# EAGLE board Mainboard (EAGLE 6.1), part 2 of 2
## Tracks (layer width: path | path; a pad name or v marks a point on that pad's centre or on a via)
!MOT0_FLAG  (via drill 0.6)
  Sig1 0.254: U$2.24 42.48,56.77 v42.86,57.15
  Sig1 0.406: U$3.31 74.36,23.88 v74.61,24.13 | v64.77,45.72 64.77,41.91 68.58,38.1 72.39,38.1 75.25,35.24 v75.25,31.11
  Sig2 0.406: v74.61,24.13 76.2,25.72 76.2,30.16 v75.25,31.11
  Bottom_GND 0.406: v42.86,57.15 42.86,49.21 43.18,48.9 60.01,48.9 62.87,46.04 64.45,46.04 v64.77,45.72
!MOT1_FLAG  (via drill 0.6)
  Sig1 0.254: U$2.23 41.39,57.27 v41.91,57.78
  Sig1 0.406: U$4.31 99.76,23.88 v100.17,24.29 | v100.01,30.8 97.79,33.02 97.79,35.56 96.2,37.15 87.95,37.15 87.63,37.47 74.93,37.47 73.03,39.37 69.22,39.37 67.31,41.27 v67.31,43.81
  Bottom_GND 0.406: v100.17,24.29 100.17,24.61 101.6,26.04 101.6,29.21 v100.01,30.8 | v41.91,57.78 41.91,49.21 42.86,48.26 59.69,48.26 62.55,45.4 63.5,45.4 64.14,44.77 66.36,44.77 v67.31,43.81
!MOT2_FLAG  (via drill 0.6)
  Sig1 0.305: U$2.16 37.21,59.75 v37.15,59.69
  Sig1 0.406: U$5.31 125.16,23.88 v125.41,24.13
  Sig2 0.406: v125.41,24.13 126.84,25.72 127,30.48 v126.36,31.11
  Bottom_GND 0.406: v37.15,59.69 37.15,49.21 41.27,45.09 58.1,45.09 61.59,41.59 86.68,41.59 90.81,37.47 95.89,37.47 100.65,32.7 106.68,32.7 107.95,31.43 126.05,31.43 v126.36,31.11
!MOT3_FLAG  (via drill 0.6)
  Sig1 0.305: U$2.15 37.71,60.72 v38.1,60.33
  Sig1 0.406: U$6.31 149.92,23.88 v150.18,24.13
  Sig2 0.406: v150.18,24.13 150.18,24.45 151.45,25.72 151.45,29.21 v148.91,31.75
  Bottom_GND 0.406: v38.1,60.33 38.1,49.21 41.59,45.72 58.42,45.72 61.91,42.23 87,42.23 91.12,38.1 96.2,38.1 100.97,33.34 107,33.34 107.63,32.7 147.96,32.7 v148.91,31.75
!MOT4_FLAG  (via drill 0.6)
  Sig1 0.305: U$2.60 49.37,58.27 v49.85,57.78
  Sig1 0.406: U$7.31 137.06,51.82 v137.48,52.23
  Bottom_GND 0.406: v49.85,57.78 49.85,57.15 56.83,50.16 60.64,50.16 63.5,47.31 65.41,47.31 66.67,46.04 66.99,46.04 67.31,45.72 67.63,45.72 69.22,44.13 87,44.13 87.95,45.09 87.95,57.78 89.53,59.37 137.79,59.37 139.06,58.1 139.06,54.93 137.48,53.34 v137.48,52.23
!MOT5_FLAG  (via drill 0.6)
  Sig1 0.305: U$2.59 48.28,57.77 v48.9,57.15
  Sig1 0.406: U$8.31 111.03,51.82 111.76,52.55 112.55,52.55 113.51,53.5 v113.82,53.5
  Bottom_GND 0.406: v48.9,57.15 56.52,49.53 60.33,49.53 63.18,46.67 65.09,46.67 66.36,45.4 66.67,45.4 66.99,45.09 67.31,45.09 68.9,43.5 87.95,43.5 88.9,44.45 88.9,48.9 89.53,49.53 92.71,49.53 93.66,50.48 93.66,51.75 96.2,54.29 112.87,54.29 v113.82,53.5
!MOT_RESET  (via drill 0.6)
  Sig1 0.406: U$3.6 56.26,23.88 v55.88,23.5 | v78.11,31.75 v81.28,31.75 | v103.82,31.75 v106.36,31.75 | v131.13,31.75 v128.59,31.75 120.33,40.01 v119.7,40.01 | U$4.6 82.3,23.88 v81.92,23.5 | U$5.6 108.01,23.88 v107.63,23.5 | U$6.6 131.83,23.88 v131.44,23.5 | U$7.6 119.92,51.82 119.38,51.28 v119.38,50.8 | U$8.6 95.31,51.82 v94.61,51.12
  Sig2 0.406: v55.88,23.5 55.88,29.84 58.1,32.07 77.79,32.07 v78.11,31.75 | v103.82,31.75 103.19,32.07 81.6,32.07 v81.28,31.75 81.28,24.13 v81.92,23.5 | v128.59,31.75 128.27,32.07 106.68,32.07 v106.36,31.75 106.36,24.77 v107.63,23.5 | v131.13,31.75 131.44,31.43 v131.44,23.5
  Bottom_GND 0.406: v119.38,50.8 119.06,50.48 117.47,50.48 115.57,48.42 115.57,43.18 | 115.57,43.18 118.75,40.01 v119.7,40.01 | v94.61,51.12 94.61,49.85 95.89,48.58 95.89,41.59 98.11,39.37 111.76,39.37 115.57,43.18
!SPI_CS  (via drill 0.6)
  Sig1 0.254: U$2.20 38.13,58.77 v39.05,59.69 | U$3.30 75.21,23.22 75.25,23.18 75.88,23.81
  Sig1 0.406: U$4.30 100.53,23.22 v101.28,24.29 | U$3.30 75.29,23.22 75.88,23.81 v75.88,24.13 | U$5.30 126.24,23.22 126.84,23.81 v126.84,24.45 | U$6.30 150.53,23.22 v151.45,24.13 | v62.55,43.18 68.26,37.47 72.07,37.47 73.66,35.88 v73.66,31.11 | U$7.30 137.76,51.16 v138.11,51.12 | v109.86,40.32 109.86,32.07 v107.63,29.84 | U$8.30 111.64,51.16 v112.08,51.59
  Bottom_GND 0.406: 107,24.45 105.73,23.18 104.14,23.18 103.03,24.29 v101.28,24.29 100.49,23.18 87.95,23.18 86.68,24.45 81.6,24.45 80.33,23.18 79.06,23.18 78.11,24.13 v75.88,24.13 75.88,25.72 76.52,26.35 76.52,28.26 v73.66,31.11 | 107,24.45 112.39,24.45 113.03,23.81 123.83,23.81 125.09,25.08 126.36,25.08 v126.84,24.45 127.64,23.81 128.27,23.81 129.86,22.23 130.49,22.23 130.81,22.54 149.86,22.54 v151.45,24.13 | v39.05,59.69 39.05,49.21 41.91,46.35 58.74,46.35 61.91,43.18 v62.55,43.18 | v138.11,51.12 136.53,51.12 135.57,52.07 135.57,56.83 134.94,57.47 123.51,57.47 122.87,58.1 117.16,58.1 115.57,56.52 115.57,53.82 113.82,52.07 112.55,52.07 v112.08,51.59 110.49,50.16 110.49,40.96 v109.86,40.32 | v107.63,29.84 107.63,25.08 107,24.45
+3V3  (via drill 0.6)
  Sig1 0.254: R57.2 32.07,13.34 32.06,13.33 R57.2 R60.2 32.06,18.09 33.66,19.68 36.2,19.68 38.73,22.23 38.73,23.5 | R57.2 R56.2 | U$19.15 35.71,29.38 37.15,27.94 C47.1 C44.1 | U$19.17 37.25,30.38 37.47,30.16 C45.1 C44.1 | U$19.21 37.48,32.38 38.1,32.38 C44.1 | U$19.28 30.36,36.72 31.11,37.47 33.34,37.47 35.24,35.56 35.88,35.56 | 35.88,35.56 36.04,35.72 C46.1 | R57.2 34.29,13.02 34.77,12.54 34.77,11.59 C55.1 | U$2.42 41.71,53.77 42.23,54.29 44.77,54.29 45.4,53.66 45.4,52.07 45.72,51.75 47.31,51.75 v47.94,51.12 | U$19.8 29.86,25.06 30.16,24.77 31.43,24.77 31.75,24.45 C48.1 | U$19.11 31.36,26.26 31.59,26.04 32.38,26.04 33.02,26.67 C49.1 | C49.1 C48.1 | C48.1 | C44.1 38.74,25.4 | 38.74,25.4 39.69,24.45 v41.91,24.45 | C49.1 34.29,23.5 34.61,23.18 38.42,23.18 38.73,23.5 | 38.73,23.5 38.73,25.4 38.74,25.4 | 35.88,35.56 35.88,36.51 36.2,36.83 45.4,36.83 v47.94,34.29 | U$19.4 27.86,28.33 v27.3,28.89 27.3,29.53 27.62,29.84 30.8,29.84 v31.43,29.21 | C12.1 | C38.1
  Sig1 0.305: C7.2 66.67,47.78 66.04,48.42 66.04,50.01 | 66.04,50.01 66.88,50.84 IC1.5 | IC1.2 67.11,52.34 66.99,52.23 65.72,52.23 65.41,51.91 65.41,51.59 65.53,51.47 | IC1.3 67.24,51.84 66.99,51.59 65.53,51.59 | 65.53,51.59 C18.+ | 65.53,51.47 66.04,50.96 66.04,50.01 | 65.53,51.59 65.53,51.47 | C43.1 | U$2.54 48.88,55.27 v48.9,55.24 | C9.1 38.73,67.63 39.71,66.66 U$2.11 39.71,60.94 41.59,59.05 v42.23,59.05 | v59.37,56.2 59.37,53.98 | v44.45,60.33 44.21,60.57 U$2.2 44.21,63.26 45.4,64.45 v45.4,65.09 | v60.33,57.15 60.33,53.98 | U$2.26 33.54,55.77 32.47,56.83 31.75,56.83 31.11,56.2 C12.1 28.26,54.93 26.35,53.02 26.35,49.53 25.72,48.9 v19.68,48.9 | U$2.37 39.21,49.05 38.42,48.26 C43.1 | C43.1 34.61,50.16 33.97,50.8 v33.02,50.8
  Sig1 0.406: U$4.24 97.09,19.3 96.84,19.05 96.84,13.97 | 96.84,13.97 96.84,12.06 | U$3.24 71.69,19.3 71.44,19.05 71.44,13.97 | 71.44,13.97 71.44,12.06 | U$5.24 122.49,19.3 122.24,19.05 122.24,13.65 | 122.24,13.65 122.24,11.75 | U$6.24 146.94,19.3 146.69,19.05 146.69,12.06 146.37,11.75 | v117.95,48.9 117.47,48.42 117.47,47.47 116.84,46.83 113.19,46.83 112.78,47.24 U$8.24 108.52,47.24 108.52,47.37 108.27,47.62 108.27,64.45 107.95,64.77 92.39,64.77 91.44,65.72 91.44,68.9 v90.49,69.85 | U$7.24 137.73,47.24 v138.11,47.62 | C24.1 71.44,13.97 | C10.1 96.84,13.97 | C13.1 122.24,13.65 | R3.1 57.47,53.98 | R39.1 57.15,53.98 | R38.1 54.93,52.7 | 54.93,52.7 56.2,53.98 55.24,54.93 v55.24,56.2 | v47.94,51.12 52.7,51.12 54.29,52.7 54.93,52.7 | C38.1 18.73,53.66 19.68,52.7 v19.68,48.9 | 126.36,81.92 v126.36,81.6 U$18.6 | U$9.6 v114.94,81.6 | U$10.6 v103.5,81.6 | U$11.6 v92.08,81.6 | U$12.6 v80.64,81.6 | U$13.6 v69.22,81.6 | U$14.6 v57.78,81.6 | U$15.6 v46.35,81.6 | U$16.6 v34.92,81.6 | U$17.6 v23.5,81.6 | v60.33,64.45 v60.33,57.15
  Sig1 0.61: IC2.16 18.73,70.48 17.78,69.53 17.78,65.09 17.14,64.45 17.14,61.28 17.78,60.64 C38.1 | U$24.6 49.21,19.68 49.53,20 | v19.68,48.9 16.19,48.9 14.29,46.99 C50.1 14.29,39.05 14.61,38.73 14.61,37.78 | 14.61,37.78 R53.1 14.61,37.78 | 14.61,37.78 13.02,37.78 12.7,37.47 v12.7,37.15 | v12.38,31.43 12.7,31.11 14.61,31.11 14.92,30.8 R41.2 | R41.2 R40.2 | R41.2 13.97,29.52 12.06,27.62 9.84,27.62 | 9.84,27.62 4.45,27.62 3.49,28.57 3.49,29.43 ACTLED.A | R42.2 9.85,27.62 9.84,27.62
  Sig1 0.813: ACTLED.A LINKLED.A SPDLED.A
  Sig1 1.016: 146.37,11.75 139.7,11.75 138.59,12.86 137,12.86 135.89,11.75 122.24,11.75 115.25,11.75 114.14,12.86 111.92,12.86 111.12,12.06 96.84,12.06 89.53,12.06 88.74,12.86 87.15,12.86 86.36,12.06 71.44,12.06 64.77,12.06 63.98,12.86 62.39,12.86 61.59,12.06 54.61,12.06 52.7,13.97 52.7,18.41 51.12,20 49.53,20 46.35,20 v41.91,24.45
  Sig1 1.27: C18.+ 63.98,51.91 63.82,51.75 | v54.61,42.23 58.74,42.23 62.87,46.35 62.87,50.8 63.82,51.75 | 63.82,51.75 63.82,53.02 62.87,53.98 60.33,53.98 59.37,53.98 57.47,53.98 57.15,53.98 56.2,53.98
  Sig2 0.305: v33.02,50.8 31.43,50.8 30.8,50.16 30.8,48.9
  Sig2 1.27: 41.91,29.21 41.91,32.07 44.13,34.29 v47.94,34.29 50.16,36.51 50.16,39.69 52.7,42.23 v54.61,42.23 54.61,46.04 51.75,48.9 30.8,48.9 v19.68,48.9 19.68,77.79 v23.5,81.6 v34.92,81.6 v46.35,81.6 v57.78,81.6 v69.22,81.6 v80.64,81.6 v92.08,81.6 v103.5,81.6 v114.94,81.6 v126.36,81.6 | 41.91,29.21 v41.91,24.45 | v31.43,29.21 41.91,29.21
  Bottom_GND 0.305: v42.23,59.05 42.55,59.37 58.42,59.37 59.37,58.42 v59.37,56.2 | v44.45,60.33 45.09,60.33 45.4,60.01 58.74,60.01 60.33,58.42 v60.33,57.15
  Bottom_GND 0.406: v117.95,48.9 118.9,49.85 121.6,49.85 124.46,46.99 137.48,46.99 v138.11,47.62 | v90.49,69.85 79.38,69.85 78.74,70.48 78.74,73.03 78.11,73.66 X29.1 76.2,73.66 75.88,73.34 75.88,69.53 74.93,68.58 62.23,68.58 60.33,66.67 v60.33,64.45
  Bottom 0.254: v27.3,28.89 24.13,28.89 23.81,28.57 C23.1 | v47.94,51.12 C22.1 | C21.1
  Bottom 0.305: v48.9,55.24 C21.1 | v45.4,65.09 45.09,65.41 C11.1
  Bottom 0.406: C21.1 51.12,56.52 51.44,56.83 54.61,56.83 v55.24,56.2
  Bottom 0.61: v12.7,37.15 12.7,36.2 | 12.7,36.2 13.02,35.88 R52.1 | v12.38,31.43 12.38,35.88 12.7,36.2
+5V
  Sig1 0.254: 72.2,51.91 72.2,51.78 72.39,51.59 | IC1.8 72.12,50.84 72.71,51.44 72.71,51.59
  Sig1 0.305: 72.39,51.59 72.71,51.59 | 72.39,52.86 72.64,52.36 | 72.64,52.36 72.71,52.23 | IC1.11 71.87,52.34 72.71,53.18 | IC1.10 71.69,51.84 71.75,51.91 72.2,51.91 72.64,52.36
  Sig1 0.406: 71.75,63.02 U$1.4 | 81.92,56.04 82.1,56.04 L1.P$2
  Sig1 0.61: 71.75,63.02 71.75,63.98 71.44,64.29 64.14,64.29 63.5,63.66 R1.1
  Sig1 1.016: C5.+ 82.55,55.4 81.92,56.04 | C6.+ 75.56,53.82 74.61,54.77
  Sig1 1.27: L1.P$2 77.92,56.17 76.52,54.77 74.61,54.77 72.07,54.77 | 72.07,54.77 71.75,54.77 71.12,55.4 D1.A 71.12,62.39 71.75,63.02 | 72.71,51.59 72.71,53.18 72.71,54.13 72.07,54.77
+24V  (via drill 0.6)
  Sig1 0.61: U$1.2 76.68,60.48 76.83,60.33
  Sig1 1.422: X1.1 4.76,47.62 8.89,51.75 10.48,51.75 10.48,51.76 C1.1 C2.1 v16.19,51.76 v16.19,51.75 | v85.72,61.28 84.45,60.01 77.15,60.01 76.83,60.33
  Bottom_GND 1.422: v16.19,51.75 27.3,62.71 84.3,62.71 v85.72,61.28
ACTLED  (via drill 0.6)
  Sig1 0.254: R51.1 12.38,29.53 v13.02,30.16 | U$19.27 30.86,36.26 31.43,36.83 33.34,36.83 35.24,34.92 v35.24,34.29
  Bottom_GND 0.254: v13.02,30.16 30.48,30.16 33.34,33.02 34.61,33.02 35.24,33.66 v35.24,34.29
DIN0
  Sig1 0.305: R27.2 120.65,83.82 119.7,82.87 119.7,80.64 114.62,75.56 45.4,75.56 44.71,74.87 44.71,68.64 46.35,66.99 46.35,64.45 44.71,62.8 U$2.1
  Sig1 0.406: R27.2 125.04,83.82 U$18.5
DIN1
  Sig1 0.305: 113.67,83.82 113.67,80.33 109.54,76.2 45.09,76.2 44.13,75.25 44.13,65.41 43.21,64.48 U$2.4
  Sig1 0.406: U$9.5 113.61,83.82 R10.2 113.67,83.82
DIN2
  Sig1 0.305: 102.23,83.5 102.23,80.33 98.74,76.83 44.77,76.83 43.5,75.56 43.5,65.72 42.71,64.93 U$2.5
  Sig1 0.406: R13.2 102.18,83.82 U$10.5 102.23,83.5
DIN3
  Sig1 0.305: 90.81,83.5 90.81,80.33 87.95,77.47 44.45,77.47 42.86,75.88 42.86,66.04 42.21,65.39 U$2.6
  Sig1 0.406: R16.2 90.75,83.82 U$11.5 90.81,83.5
DIN4
  Sig1 0.305: U$12.5 79.38,80.33 77.15,78.11 44.13,78.11 42.23,76.2 42.23,66.36 41.71,65.84 U$2.7
  Sig1 0.406: R19.2 79.32,83.82 U$12.5
DIN5
  Sig1 0.305: U$13.5 67.94,80.33 66.36,78.74 43.81,78.74 41.59,76.52 41.59,66.67 41.21,66.29 U$2.8
  Sig1 0.406: R22.2 67.89,83.82 U$13.5
DIN6
  Sig1 0.305: U$14.5 56.52,80.33 55.56,79.38 43.5,79.38 40.96,76.83 40.96,66.99 40.71,66.74 U$2.9
  Sig1 0.406: R25.2 56.46,83.82 U$14.5
DIN7
  Sig1 0.305: U$15.5 45.09,80.64 44.45,80.01 43.18,80.01 40.32,77.15 40.32,67.31 40.21,67.19 U$2.10
  Sig1 0.406: R30.2 45.03,83.82 U$15.5
DIN8
  Sig1 0.305: U$16.5 33.66,80.64 34.92,79.38 37.47,79.38 39.69,77.15 39.69,74.3 37.15,71.75 37.15,66.36 38.71,64.8 U$2.13
  Sig1 0.406: U$16.5 31.49,83.76 R33.2
DIN9
  Sig1 0.305: U$17.5 22.23,80.64 24.13,78.74 37.15,78.74 39.05,76.83 39.05,74.61 36.51,72.07 36.51,66.04 38.21,64.34 U$2.14
  Sig1 0.406: U$17.5 20.06,83.76 R36.2
DISP_CLK
  Sig1 0.305: U$2.61 48.92,58.77 49.85,59.69 49.85,67.15 49.53,67.47 49.53,71.44 50.48,72.39 81.28,72.39 X29.5
DISP_CS  (via drill 0.6)
  Sig1 0.305: U$2.62 48.47,59.27 49.21,60.01 49.21,66.99 48.9,67.31 48.9,71.75 50.48,73.34 v67.94,73.34 | v84.45,71.12 X29.6
  Bottom_GND 0.305: v67.94,73.34 69.53,74.93 84.14,74.93 85.09,73.98 85.09,71.75 v84.45,71.12
DISP_SDI  (via drill 0.6)
  Sig1 0.305: U$2.63 48.02,59.77 48.58,60.33 48.58,66.67 48.26,66.99 48.26,72.07 50.16,73.98 67.31,73.98 67.63,74.3 69.53,74.3 69.85,73.98 v69.85,73.34 | v74.93,69.85 78.74,69.85 X29.4
  Bottom_GND 0.305: v69.85,73.34 70.48,73.34 73.98,69.85 v74.93,69.85
DISP_SDO
  Sig1 0.305: U$2.64 47.56,60.27 47.94,60.64 47.94,66.36 47.62,66.67 47.62,72.39 49.85,74.61 66.99,74.61 67.31,74.93 79.69,74.93 80.01,74.61 X29.3
ETH_!INT  (via drill 0.6)
  Sig1 0.254: R53.2 25.72,37.47 26.36,36.82 U$19.36 26.36,33.64 v26.67,33.34 | U$2.43 42.21,52.69 42.86,53.34 v44.13,53.34
  Bottom 0.254: v44.13,53.34 44.13,33.66 43.5,33.02 26.99,33.02 v26.67,33.34
ETH_CLK
  Sig1 0.254: U$19.33 27.86,52.63 29,53.77 U$2.30
ETH_CS
  Sig1 0.254: U$19.32 28.36,52.49 29.14,53.27 U$2.31
ETH_SDI
  Sig1 0.254: U$19.35 26.86,52.9 28.73,54.77 U$2.28
ETH_SDO
  Sig1 0.254: U$19.34 27.36,52.77 28.86,54.27 U$2.29
GND  (via drill 0.6)
  Sig1 0.254: U$2.39 40.21,49.59 39.69,49.07 39.69,48.9 37.31,46.51 36.35,46.51 | U$2.35 38.21,49.5
  Sig1 0.305: U$2.3 43.71,63.87 v44.29,64.45 | U$2.12 39.21,65.57 38.42,66.36 v38.58,66.36 | v32.07,55.56 32.38,55.24 35.24,55.24 35.24,55.25 U$2.27 | U$2.55 47.83,55.77 v48.26,56.2
  other vias: 3.17,3.17 9.53,3.17 15.88,3.17 22.23,3.17 28.57,3.17 34.92,3.17 41.27,3.17 41.27,9.53 41.27,15.88 41.27,22.23 3.17,9.53 3.17,15.88 3.17,22.23 3.17,38.1 3.17,44.45 3.17,50.8 19.05,41.27 22.23,50.8 22.23,53.98 3.17,57.15 3.17,63.5 3.17,69.85 31.75,73.03 3.17,76.2 3.17,82.55 3.17,88.9 3.17,95.25 9.53,95.25 15.88,95.25 15.88,88.27 47.62,38.1 69.85,79.38 82.55,79.38 92.08,79.38 104.78,79.38 120.65,76.2 127,76.2 133.35,76.2 92.71,71.12 99.06,71.12 104.14,71.12 109.22,71.12 114.3,71.12 119.38,71.12 124.46,71.12 129.54,71.12 134.62,71.12 139.7,71.12 139.7,77.47 139.7,82.55 139.7,87.63 139.7,92.71 139.7,97.79 142.24,97.79 147.32,97.79 152.4,97.79 157.48,97.79 157.48,93.98 157.48,88.9 157.48,83.82 157.48,78.74 157.48,72.39 157.48,67.31 157.48,60.96 157.48,55.88 157.48,50.8 157.48,45.72 157.48,39.37 157.48,32.7 157.48,29.21 157.48,24.13 157.48,19.05 157.48,13.97 157.48,8.89 157.48,3.81 156.21,2.54 153.67,2.54 147.32,2.54 140.97,2.54 134.62,2.54 125.73,2.54 120.65,2.54 114.3,2.54 109.22,2.54 104.14,2.54 97.79,2.54 92.71,2.54 86.36,2.54 81.28,2.54 76.2,2.54 71.12,2.54 64.77,2.54 59.69,2.54 54.61,2.54 49.53,2.54 45.72,25.4 45.72,30.48 62.23,29.21 62.23,27.3 62.23,25.4 62.23,23.5 62.23,21.59 62.23,19.68 62.23,17.46 62.23,14.92 70.48,27.3 70.48,25.4 70.48,23.5 70.48,21.59 70.48,19.68 70.48,17.46 70.48,14.92 87.63,29.21 87.63,27.3 87.63,25.4 87.63,17.46 87.63,14.92 95.89,27.3 95.89,25.4 95.89,17.46 95.89,14.92 113.03,29.21 121.28,29.21 113.03,27.3 121.28,27.3 113.03,25.4 121.28,25.4 113.03,21.59 121.28,21.59 113.03,17.46 113.03,14.92 121.28,17.46 121.28,14.92 137.48,14.92 137.48,17.46 137.48,23.5 137.48,25.4 137.48,27.3 137.48,29.21 145.73,27.3 145.73,25.4 145.73,23.5 145.73,19.68 145.73,17.46 145.73,14.92 99.06,57.15 99.06,55.24 99.06,53.34 99.06,49.53 107.31,57.15 107.31,55.24 107.31,53.34 107.31,49.53 107.31,45.4 107.31,42.86 99.06,45.4 99.06,42.86 123.83,42.86 123.83,45.4 123.83,51.44 123.83,53.34 123.83,55.24 132.08,55.24 132.08,53.34 132.08,51.44 132.08,45.4 132.08,42.86 25.08,75.25 39.05,72.39 33.02,52.07 36.26,46.45 33.66,34.92 73.03,14.92 98.42,14.92 124.14,14.61 119.38,48.74 94.77,48.42 113.35,51.12 90.33,40.64 81.44,40.01 55.56,60.96 58.26,52.55 66.83,61.28 87,53.5 87,50.96
  pour Bottom: 45.72,0.95 157.16,0.95 159.07,2.86 159.07,97.79 157.8,99.06 139.38,99.06 138.11,97.79 138.11,74.93 136.21,73.03 91.12,73.03 89.85,71.75 89.85,42.55 87.95,40.64 53.66,40.64 52.07,39.05 52.07,33.66 50.8,32.38 45.09,32.38 43.81,31.11 43.81,2.86
  cutout Bottom_GND: 45.72,0.95 157.16,0.95 159.07,2.86 159.07,97.79 157.8,99.06 139.38,99.06 138.11,97.79 138.11,74.93 136.21,73.03 91.12,73.03 89.85,71.75 89.85,42.55 87.95,40.64 53.66,40.64 52.07,39.05 52.07,33.66 50.8,32.38 45.09,32.38 43.81,31.11 43.81,2.86
  pour Sig1: 45.72,0.95 157.16,0.95 159.07,2.86 159.07,97.79 157.8,99.06 139.38,99.06 138.11,97.79 138.11,74.93 136.21,73.03 91.12,73.03 89.85,71.75 89.85,42.55 87.95,40.64 53.66,40.64 52.07,39.05 52.07,33.66 50.8,32.38 45.09,32.38 43.81,31.11 43.81,2.86
  pour Bottom: 43.18,2.86 41.27,0.95 2.86,0.95 0.95,2.86 0.95,97.79 2.22,99.06 16.83,99.06 18.1,97.79 18.1,87.31 20,85.41 135.89,85.41 137.48,83.82 137.48,75.25 135.89,73.66 90.81,73.66 89.22,72.07 89.22,42.86 87.63,41.27 53.34,41.27 51.44,39.37 51.44,33.97 50.48,33.02 44.77,33.02 43.18,31.43
  cutout Bottom_GND: 43.18,2.86 41.27,0.95 2.86,0.95 0.95,2.86 0.95,97.79 2.22,99.06 16.83,99.06 18.1,97.79 18.1,87.31 20,85.41 135.89,85.41 137.48,83.82 137.48,75.25 135.89,73.66 90.81,73.66 89.22,72.07 89.22,42.86 87.63,41.27 53.34,41.27 51.44,39.37 51.44,33.97 50.48,33.02 44.77,33.02 43.18,31.43
  cutout Sig2: 43.18,2.86 41.27,0.95 2.86,0.95 0.95,2.86 0.95,97.79 2.22,99.06 16.83,99.06 18.1,97.79 18.1,87.31 20,85.41 135.89,85.41 137.48,83.82 137.48,75.25 135.89,73.66 90.81,73.66 89.22,72.07 89.22,42.86 87.63,41.27 53.34,41.27 51.44,39.37 51.44,33.97 50.48,33.02 44.77,33.02 43.18,31.43
  pour Sig1: 43.18,2.86 41.27,0.95 2.86,0.95 0.95,2.86 0.95,97.79 2.22,99.06 16.83,99.06 18.1,97.79 18.1,87.31 20,85.41 135.89,85.41 137.48,83.82 137.48,75.25 135.89,73.66 90.81,73.66 89.22,72.07 89.22,42.86 87.63,41.27 53.34,41.27 51.44,39.37 51.44,33.97 50.48,33.02 44.77,33.02 43.18,31.43
  cutout Sig2: 45.72,0.95 157.16,0.95 159.07,2.86 159.07,97.79 157.8,99.06 139.38,99.06 138.11,97.79 138.11,74.93 136.21,73.03 91.12,73.03 89.85,71.75 89.85,42.55 87.95,40.64 53.66,40.64 52.07,39.05 52.07,33.66 50.8,32.38 45.09,32.38 43.81,31.11 43.81,2.86
GND@5
  Bottom 0.406: R4.1 R7.1 47.31,4.76 X2.1
GNDINT  (via drill 0.6)
  Sig1 0.406: U$24.2 47.94,9.84 48.58,9.21 53.34,9.21 53.66,8.89 v53.66,6.03
  Bottom 0.406: X2.2 53.02,4.45 53.66,5.08 v53.66,6.03 53.66,8.07 C72.1 53.34,8.26
HARDSTOP  (via drill 0.6)
  Sig1 0.406: U$5.7 108.94,23.22 107.31,21.59 v106.68,21.59 | U$3.7 57.19,23.22 v56.2,22.23 | v131.44,21.59 131.76,21.59 133.39,23.22 U$6.7 136.25,23.22 136.53,23.5 136.53,30.16 133.99,32.7 130.81,32.7 122.87,40.64 122.87,50.8 122.52,51.16 U$7.7 | U$4.7 83.86,23.22 82.55,21.91 v81.28,21.91 | U$8.7 97.75,51.16 98.11,50.8 98.11,36.2 98.42,35.88 98.42,33.34 100.01,31.75 101.92,31.75 102.55,31.11 v102.55,30.16 | U$24.5 v50.48,14.61
  Sig2 0.406: v101.6,23.02 102.23,23.65 102.23,28.89 102.55,29.21 v102.55,30.16
  Bottom_GND 0.406: v131.44,21.59 129.54,21.59 127.95,23.18 108.9,23.18 107.31,21.59 v106.68,21.59 106.05,21.59 105.09,22.54 102.08,22.54 v101.6,23.02 101.12,22.54 82.55,22.54 81.92,21.91 v81.28,21.91 80.96,21.91 80.33,22.54 56.52,22.54 v56.2,22.23 56.2,20.64 55.56,20 54.29,20 50.48,16.19 v50.48,14.61
  Bottom 0.406: v50.48,14.61 R5.2
IGND  (via drill 0.6)
  other vias: 20.32,92.71 20.32,97.16 20.32,88.27 135.89,97.16 135.89,92.71 135.89,88.27
  pour Sig1: 19.05,97.79 19.05,87.63 20.32,86.36 135.89,86.36 137.16,87.63 137.16,97.79 135.89,99.06 20.32,99.06
  pour Bottom: 19.05,97.79 19.05,87.63 20.32,86.36 135.89,86.36 137.16,87.63 137.16,97.79 135.89,99.06 20.32,99.06
JTAG_!RST  (via drill 0.6)
  Sig1 0.254: 55.56,67.94 X15.5 56.83,67.94 57.47,67.31 C17.1 58.42,63.18 58.74,62.87 58.74,59.05 58.42,58.74 R3.2
  Sig1 0.305: U$2.38 39.71,53.99 40.96,55.24 v44.77,55.24 | v55.56,58.58 56.2,58.58 56.36,58.74 R3.2
  Bottom_GND 0.305: v44.77,55.24 44.77,57.47 46.04,58.74 54.77,58.74 54.93,58.58 v55.56,58.58
JTAG_TCK
  Sig1 0.305: X15.1 50.64,55.4 49.5,54.27 U$2.52
JTAG_TDI
  Sig1 0.254: 53.02,67.63 X15.3
  Sig1 0.305: U$2.50 51.36,53.27 53.02,54.93 53.02,67.63
JTAG_TDO
  Sig1 0.305: X15.4 53.34,70.48 54.29,69.53 54.29,53.98 53.08,52.77 U$2.49
JTAG_TMS
  Sig1 0.305: U$2.51 50.27,53.77 51.75,55.24 51.75,69.37 X15.2
LINKLED  (via drill 0.6)
  Sig1 0.254: R50.1 13.18,32.38 v13.34,32.54 | v32.7,35.88 32.38,36.2 32.07,36.2 31.86,35.99 U$19.25
  Bottom_GND 0.254: v13.34,32.54 29.37,32.54 v32.7,35.88
N$1
  Sig1 0.406: U$1.8 68.84,58.2 68.58,57.94 68.58,57.15 C3.1 68.58,56.67
N$2  (via drill 0.6)
  Sig1 0.406: 82.23,66.04 86.36,66.04 87,66.67 87,67.63 86.36,68.26 v85.72,68.26
  Sig1 0.61: U$1.3 78.11,61.75
  Sig1 1.27: 78.11,61.75 80.64,61.75 82.23,63.34 82.23,65.88 | 82.23,65.88 82.23,66.04 L1.P$1 | D2.C 74.3,68.1 76.52,65.88 82.23,65.88
  Bottom 0.406: v85.72,68.26 81.12,68.26 C4.2
N$3  (via drill 0.6)
  Sig1 0.406: D1.C 76.2,56.99 76.83,57.63 | 76.83,57.63 76.83,58.58 76.2,59.21 U$1.1 73.98,59.21 | v78.42,57.94 78.11,57.63 76.83,57.63
  Bottom 0.406: v78.42,57.94 78.42,58.9 77.15,60.17 74.3,60.17 73.66,60.8 73.66,66.04 75.09,67.47 75.56,67.47 75.88,67.79 75.88,68.26 v76.04,68.42 C4.1 | C4.1 | C4.1 79.06,68.26
N$4
  Sig1 0.305: U$2.48 44.71,49.91 45.09,49.53 51.44,49.53 53.66,47.31 53.66,44.77 53.98,44.45 54.83,44.45 LED1.C
N$5
  Sig1 0.305: C19.1 48.26,41.91 49.53,43.18 49.53,44.7 Q1.2 48.01,46.35 41.59,46.35 41.21,46.74 U$2.41
N$6
  Sig1 0.305: C20.1 41.27,41.91 40.01,43.18 40.01,44.7 Q1.1 40.01,44.83 40.01,46.04 40.71,46.74 U$2.40
N$7
  Sig1 0.254: R1.2 65.72,59.85
  Sig1 0.61: U$1.7 67.31,60.48 66.67,59.85 65.72,59.85 R1.2 | R1.2 R2.1
N$8
  Sig1 0.305: C7.1 70.48,48.42 69.85,49.05 66.99,49.05 66.83,49.21 66.83,50.01 67.15,50.32 67.75,50.32 IC1.6
N$9  (via drill 0.6)
  Sig1 0.406: U$4.27 100.32,21.26 v100.81,21.27 | U$3.25 74.33,19.96 74.93,19.37 76.52,19.37 76.83,19.68 v76.83,21.59
  Bottom_GND 0.406: v76.83,21.59 80.01,21.59 80.64,20.95 81.92,20.95 82.55,21.59 v100.81,21.27
N$10
  Sig1 0.406: U$6.25 151.09,19.96 152.4,21.27 153.35,21.27 154.62,22.54 154.62,27.62 152.4,29.84 152.4,36.83 151.45,37.78 146.37,37.78 144.78,39.37 144.78,48.9 142.88,50.8 139.38,50.8 138.75,50.16 136.84,50.16 135.88,49.2 U$7.27
N$11  (via drill 0.6)
  Sig1 0.406: U$3.13 57.53,19.3 v57.15,19.68 | v70.8,30.48 C26.1
  Sig2 0.406: v57.15,19.68 57.47,19.37 59.37,19.37 59.69,19.68 59.69,30.48 60.64,31.43 69.85,31.43 v70.8,30.48
N$12  (via drill 0.6)
  Sig1 0.406: D3.2 C27.2 v63.18,30.48 | U$3.14 56.26,18.67 v55.88,19.05
  Sig2 0.406: v55.88,19.05 56.2,18.73 59.69,18.73 60.33,19.37 60.33,29.53 61.28,30.48 v63.18,30.48
N$13
  Sig1 0.406: D3.3 68.9,33.97 69.22,34.29 69.22,34.61 69.53,34.92 C26.2
N$14  (via drill 0.6)
  Sig1 0.406: v95.57,30.48 C28.1 | U$4.13 83.88,19.3 v82.87,20.32
  Sig2 0.406: v95.57,30.48 94.61,31.43 86.04,31.43 85.09,30.48 85.09,19.68 84.77,19.37 83.82,19.37 v82.87,20.32
N$15  (via drill 0.6)
  Sig1 0.406: D4.2 C29.2 v87.95,30.48 | U$4.14 81.98,18.67 v81.6,19.05
  Sig2 0.406: v81.6,19.05 81.92,18.73 85.09,18.73 85.72,19.37 85.72,29.53 86.68,30.48 v87.95,30.48
N$16  (via drill 0.6)
  Sig1 0.406: U$4.25 99.73,19.96 100.33,19.37 101.92,19.37 102.23,19.68 v102.23,21.27 | U$5.27 125.56,21.26 v125.73,21.27
  Bottom_GND 0.406: v102.23,21.27 104.78,21.27 105.41,20.64 108.58,20.64 108.9,20.32 124.78,20.32 v125.73,21.27
N$17
  Sig1 0.406: D4.3 93.66,33.97 93.98,34.29 93.98,34.61 94.3,34.92 94.61,34.92 C28.2
N$18  (via drill 0.6)
  Sig1 0.406: U$3.2 53.45,26.47 v53.02,26.04 | U$3.3 54.06,25.81 v53.02,24.77
  Sig1 1.27: v58.1,8.89 X3.1
  Sig2 1.27: v53.02,26.04 v53.02,24.77 53.02,13.97 v58.1,8.89
N$19  (via drill 0.6)
  Sig1 0.406: U$3.35 74.89,26.47 v75.09,26.67 | U$3.36 74.12,27.13 v75.09,28.1
  Sig1 1.27: X3.2 v63.18,11.43
  Sig2 1.27: v63.18,11.43 63.18,12.7 66.36,12.7 67.94,14.29 67.94,26.99 70.17,29.21 73.98,29.21 v75.09,28.1 v75.09,26.67
N$20  (via drill 0.6)
  Sig1 0.406: U$3.18 56.38,16.05 v54.93,14.61 | U$3.17 55.77,16.71 v54.93,15.88
  Sig1 1.27: X4.1 v69.53,9.84
  Sig2 1.27: v69.53,9.84 59.69,9.84 v54.93,14.61 v54.93,15.88
N$21  (via drill 0.6)
  Sig1 0.406: U$3.20 74.73,16.71 v75.88,15.56 | U$3.21 75.34,17.37 v75.88,16.83
  Sig1 1.27: X4.2 v74.61,9.84
  Sig2 1.27: v74.61,9.84 75.88,11.75 v75.88,15.56 v75.88,16.83
N$22  (via drill 0.6)
  Sig1 0.406: U$4.2 83.39,26.47 82.87,26.99 78.42,26.99 v78.11,26.67 | U$4.3 83.1,25.81 82.55,26.35 79.06,26.35 v78.11,25.4
  Sig1 1.27: X5.1 v82.87,8.89
  Sig2 1.27: v82.87,8.89 78.11,13.97 v78.11,25.4 v78.11,26.67
N$23  (via drill 0.6)
  Sig1 0.406: U$4.36 99.83,27.13 v100.65,27.94 | U$4.35 100.44,26.47 v100.65,26.67
  Sig1 1.27: X5.2 v87.95,11.43
  Sig2 1.27: v87.95,11.43 89.22,12.7 91.76,12.7 93.34,14.29 93.34,26.67 95.57,28.89 99.69,28.89 v100.65,27.94 v100.65,26.67
N$24  (via drill 0.6)
  Sig1 0.406: U$4.18 83.05,16.05 v81.6,14.61 | U$4.17 82.44,16.71 v81.6,15.88
  Sig1 1.27: X6.1 v94.3,9.84
  Sig2 1.27: v94.3,9.84 86.36,9.84 v81.6,14.61 v81.6,15.88
N$25  (via drill 0.6)
  Sig1 0.406: U$4.20 100.76,16.71 v101.92,15.56 | U$4.21 101.51,17.37 v101.92,16.83
  Sig1 1.27: X6.2 v99.38,9.84
  Sig2 1.27: v99.38,9.84 101.92,12.38 v101.92,15.56 v101.92,16.83
N$26
  Sig1 0.61: C40.1 23.18,61.6 22.54,62.23 IC2.4
N$27  (via drill 0.6)
  Sig1 0.406: D5.2 C31.2 v113.35,30.48 | D5.2 115.89,33.34 115.57,33.34 D5.2 | U$5.14 108.49,18.67 v108.27,18.89
  Sig2 0.406: v108.27,18.89 108.43,18.73 110.49,18.73 111.12,19.37 111.12,29.53 112.08,30.48 v113.35,30.48
N$28
  Sig1 0.406: D5.3 119.06,34.29 119.38,34.61 119.38,34.92 119.7,35.24 C30.2
N$29  (via drill 0.6)
  Sig1 0.406: v120.97,30.48 C30.1 | U$5.13 109.28,19.3 108.58,20 107.95,20 v107,19.05
  Sig2 0.406: v120.97,30.48 120.02,31.43 112.08,31.43 110.49,29.84 110.49,19.68 110.17,19.37 109.22,19.37 108.58,20 107.95,20 v107,19.05
N$30  (via drill 0.6)
  Sig1 0.406: U$5.2 109.11,26.47 108.58,26.99 104.14,26.99 v103.5,26.35 | U$5.3 108.81,25.81 108.27,26.35 104.78,26.35 v103.5,25.08
  Sig1 1.27: X7.1 v107.63,9.53
  Sig2 1.27: v107.63,9.53 103.5,13.97 v103.5,25.08 v103.5,26.35
N$31  (via drill 0.6)
  Sig1 0.406: U$5.35 125.53,26.47 v125.73,26.67 | U$5.36 124.92,27.13 v125.73,27.94
  Sig1 1.27: X7.2 v112.71,11.43
  Sig2 1.27: v112.71,11.43 121.6,11.43 122.87,12.7 122.87,23.5 125.73,26.35 v125.73,26.67 v125.73,27.94
N$32  (via drill 0.6)
  Sig1 0.406: U$5.18 108.44,16.05 v107,14.61 | U$5.17 107.84,16.71 v107,15.88
  Sig1 1.27: X8.1 v119.06,9.53
  Sig2 1.27: v119.06,9.53 112.08,9.53 v107,14.61 v107,15.88
N$33  (via drill 0.6)
  Sig1 0.406: U$5.20 125.53,16.71 v126.68,15.56 | U$5.21 126.28,17.37 v126.68,16.83
  Sig1 1.27: X8.2 v124.14,9.53
  Sig2 1.27: v124.14,9.53 126.68,11.43 v126.68,15.56 v126.68,16.83
N$34  (via drill 0.6)
  Sig1 0.406: U$8.27 111.91,49.2 v112.24,49.53 | U$7.25 137.12,47.9 138.11,48.9 140.97,48.9 v141.29,49.21
  Bottom_GND 0.406: v112.24,49.53 112.71,49.05 115.09,49.05 117.79,51.75 120.49,51.75 123.98,48.26 132.4,48.26 132.72,47.94 137.16,47.94 138.11,48.9 140.97,48.9 v141.29,49.21
N$35  (via drill 0.6)
  Sig1 0.406: v145.41,30.48 C32.1 | U$6.13 133.41,19.3 132.72,20 132.08,20 131.29,19.21 v131.29,19.05
  Sig2 0.406: v145.41,30.48 144.46,31.43 136.53,31.43 134.94,29.84 134.94,20 134.3,19.37 133.35,19.37 132.72,20 132.08,20 131.29,19.21 v131.29,19.05
N$36  (via drill 0.6)
  Sig1 0.406: D6.2 C33.2 v137.79,30.48 | U$6.14 132.78,18.67 v132.56,18.89
  Sig2 0.406: v132.56,18.89 132.72,18.73 134.94,18.73 135.57,19.37 135.57,29.53 136.53,30.48 v137.79,30.48
N$37
  Sig1 0.406: D6.3 143.51,34.29 143.83,34.61 143.83,34.92 144.15,35.24 C32.2
N$38  (via drill 0.6)
  Sig1 0.406: D7.2 C35.2 v124.14,58.42 | U$7.14 118.49,46.61 v118.27,46.83
  Sig2 0.406: v118.27,46.83 118.43,46.67 121.28,46.67 121.92,47.31 121.92,55.24 121.13,56.04 117.47,56.04 116.84,56.67 116.84,57.47 117.79,58.42 v124.14,58.42
N$39
  Sig1 0.406: D7.3 129.86,61.91 130.18,62.23 130.18,62.55 130.49,62.87 C34.2
N$40  (via drill 0.6)
  Sig1 0.406: U$7.13 119.28,47.24 v118.59,47.94 | v131.76,58.42 C34.1
  Sig2 0.406: v131.76,58.42 130.81,59.37 117.79,59.37 116.2,57.78 116.2,56.52 117.32,55.4 120.81,55.4 121.28,54.93 121.28,47.62 120.97,47.31 119.22,47.31 v118.59,47.94
N$41  (via drill 0.6)
  Sig1 0.406: U$6.2 128.7,26.47 v128.27,26.04 | U$6.3 129.31,25.81 v128.27,24.77
  Sig1 1.27: X9.1 v132.72,9.53
  Sig2 1.27: v132.72,9.53 128.27,13.97 v128.27,24.77 v128.27,26.04
N$42  (via drill 0.6)
  Sig1 0.406: U$6.35 149.97,26.47 v150.18,26.67 | U$6.36 149.37,27.13 v150.18,27.94
  Sig1 1.27: X9.2 v137.79,11.43
  Sig2 1.27: v137.79,11.43 139.06,12.7 141.6,12.7 143.19,14.29 143.19,26.99 145.1,28.89 149.22,28.89 v150.18,27.94 v150.18,26.67
N$43  (via drill 0.6)
  Sig1 0.406: U$6.18 132.57,16.05 v131.44,14.92 | U$6.17 131.97,16.71 v131.44,16.19
  Sig1 1.27: X10.1 v144.15,9.53
  Sig2 1.27: v144.15,9.53 136.84,9.53 v131.44,14.92 v131.44,16.19
N$44  (via drill 0.6)
  Sig1 0.406: U$6.20 149.97,16.71 v151.13,15.56 | U$6.21 150.41,17.37 v151.13,16.83
  Sig1 1.27: X10.2 v149.22,9.53
  Sig2 1.27: v149.22,9.53 151.13,11.43 v151.13,15.56 v151.13,16.83
N$45  (via drill 0.6)
  Sig1 0.406: U$7.2 119.9,54.41 119.38,54.93 v119.38,57.15 | U$7.3 118.97,53.75 118.11,54.61 v118.11,57.15
  Sig1 1.27: X11.1 v148.59,43.18
  Sig2 1.27: v148.59,43.18 135.25,43.18 134.3,44.13 134.3,56.2 133.35,57.15 v119.38,57.15 v118.11,57.15
N$46  (via drill 0.6)
  Sig1 0.406: U$7.36 136.03,55.07 v136.84,55.88 | U$7.35 136.64,54.41 v138.11,55.88
  Sig1 1.27: X11.2 v146.69,48.26
  Sig2 1.27: v146.69,48.26 146.69,54.61 145.41,55.88 v138.11,55.88 v136.84,55.88
N$47  (via drill 0.6)
  Sig1 0.406: U$7.18 119.88,43.99 v118.75,42.86 | U$7.17 119.27,44.65 v118.75,44.13
  Sig1 1.27: X12.1 v150.18,54.61
  Sig2 1.27: v150.18,54.61 150.18,42.55 148.91,41.27 120.33,41.27 v118.75,42.86 v118.75,44.13
N$48  (via drill 0.6)
  Sig1 0.406: U$7.21 140.56,45.31 v141.29,46.04 | U$7.20 141.17,44.65 v141.29,44.77
  Sig1 1.27: X12.2 v148.59,59.69
  Sig2 1.27: v148.59,59.69 148.59,47.62 147.64,46.67 141.6,46.67 v141.29,46.04 v141.29,44.77
N$49
  Sig1 0.61: C39.2 20.64,65.08 21.27,65.72 IC2.3
N$50  (via drill 0.6)
  Sig1 0.406: D8.2 C37.2 v99.38,58.42 | U$8.14 93.89,46.61 v93.66,46.83
  Sig2 0.406: v93.66,46.83 93.82,46.67 96.52,46.67 97.16,47.31 97.16,57.47 98.11,58.42 v99.38,58.42
N$51
  Sig1 0.406: D8.3 105.09,61.91 105.41,62.23 105.41,62.55 105.73,62.87 C36.2
N$52  (via drill 0.6)
  Sig1 0.406: v107,58.42 C36.1 | U$8.13 94.68,47.24 v93.66,48.26
  Sig2 0.406: v107,58.42 106.05,59.37 98.11,59.37 96.52,57.78 96.52,47.62 96.2,47.31 94.61,47.31 v93.66,48.26
N$53  (via drill 0.6)
  Sig1 0.406: U$8.3 92.96,53.75 v92.39,54.29 | U$8.2 93.55,54.41 v92.39,55.56
  Sig1 1.27: X13.1 v146.69,66.04
  Sig2 1.27: v146.69,66.04 94.61,66.04 92.39,63.82 v92.39,55.56 v92.39,54.29
N$54  (via drill 0.6)
  Sig1 0.406: U$8.36 110.79,55.07 v112.71,56.99 | v112.71,55.72 111.4,54.41 U$8.35
  Sig1 1.27: X13.2 v148.27,71.12
  Sig2 1.27: v148.27,71.12 148.27,65.41 147.32,64.45 115.25,64.45 112.71,61.91 v112.71,56.99 v112.71,55.72
N$55  (via drill 0.6)
  Sig1 0.406: U$8.18 90.98,43.99 v90.81,43.81 | U$8.17 91.4,44.65 v90.81,45.09
  Sig1 1.27: X14.1 v146.69,77.47
  Sig2 1.27: v146.69,77.47 146.69,68.58 145.73,67.63 93.98,67.63 90.81,64.45 v90.81,45.09 v90.81,43.81
N$56  (via drill 0.6)
  Sig1 0.406: U$8.21 111.83,45.31 v113.35,43.81 | U$8.20 111.4,44.65 v113.35,42.7
  Sig1 1.27: X14.2 v149.86,82.55
  Sig2 1.27: v149.86,82.55 149.86,64.77 147.96,62.87 115.89,62.87 114.3,61.28 114.3,55.24 115.09,54.29 115.09,47.78 113.35,46.04 v113.35,43.81 v113.35,42.7
N$57
  Sig1 0.61: C42.1 26.35,64.45 25.08,65.72 IC2.6
N$58
  Sig1 0.406: C41.1
  Sig1 0.61: IC2.2 20,68.58 20.32,68.9 30.16,68.9 30.48,68.58 C41.1
N$59
  Sig1 0.61: IC2.5 C40.2
N$60
  Sig1 0.61: IC2.1 C39.1
N$61  (via drill 0.6)
  Sig1 0.406: R26.2 R6.2 129.22,87.31 128.91,87.63 U$18.1 128.91,91.44 128.27,92.08 v125.73,92.08
  Bottom 0.406: v125.73,92.08 C56.2
N$62
  Sig1 0.406: R38.2 LED1.A
N$63  (via drill 0.6)
  Sig1 0.406: v133.35,92.08 R26.1 R6.1
  Bottom 0.406: X17.1 132.08,93.34 132.4,93.03 133.03,93.03 133.35,92.71 v133.35,92.08
N$64  (via drill 0.6)
  Sig1 0.406: v121.92,92.08 R9.1 R11.1
  Bottom 0.406: X18.1 120.65,93.66 120.97,93.34 121.6,93.34 121.92,93.03 v121.92,92.08
N$65  (via drill 0.6)
  Sig1 0.406: R9.2 R11.2 117.79,87.31 117.47,87.63 U$9.1 117.47,91.44 116.84,92.08 v114.3,92.08
  Bottom 0.406: v114.3,92.08 C61.2
N$66
  Sig1 0.406: R39.2 LED2.A
N$67  (via drill 0.6)
  Sig1 0.406: v110.49,92.08 R12.1 R14.1
  Bottom 0.406: X19.1 109.22,93.66 109.54,93.34 110.17,93.34 110.49,93.03 v110.49,92.08
N$68  (via drill 0.6)
  Sig1 0.406: R12.2 R14.2 106.36,87.31 106.05,87.63 U$10.1 106.05,91.44 105.41,92.08 v102.87,92.08
  Bottom 0.406: v102.87,92.08 C62.2
N$69
  Sig1 0.305: LED2.C 57.15,43.5 56.83,43.18 53.66,43.18 53.02,43.81 53.02,46.99 51.12,48.9 44.77,48.9 44.21,49.45 U$2.47
N$70  (via drill 0.6)
  Sig1 0.406: v99.06,92.08 R15.1 R17.1
  Bottom 0.406: X20.1 97.79,93.66 98.11,93.34 98.74,93.34 99.06,93.03 v99.06,92.08
N$71  (via drill 0.6)
  Sig1 0.406: R15.2 R17.2 94.93,87.31 94.61,87.63 U$11.1 94.61,91.44 93.98,92.08 v91.44,92.08
  Bottom 0.406: v91.44,92.08 C57.2
N$72
  Sig1 0.254: U$19.23 36.23,33.38 36.83,33.97 40.01,33.97 40.64,34.61 R43.1
N$73  (via drill 0.6)
  Sig1 0.406: v87.63,92.08 R18.1 R20.1
  Bottom 0.406: X21.1 86.36,93.66 86.68,93.34 87.31,93.34 87.63,93.03 v87.63,92.08
N$74  (via drill 0.6)
  Sig1 0.406: R18.2 R20.2 83.5,87.31 83.19,87.63 U$12.1 83.19,91.44 82.55,92.08 v80.01,92.08
  Bottom 0.406: v80.01,92.08 C60.2
N$75  (via drill 0.6)
  Sig1 0.254: U$19.38 19.01,33.38 v18.73,33.66
  Bottom 0.254: R44.1 v18.73,33.66
N$76  (via drill 0.6)
  Sig1 0.406: v76.2,92.08 R21.1 R23.1
  Bottom 0.406: X22.1 74.93,93.66 75.25,93.34 75.88,93.34 76.2,93.03 v76.2,92.08
N$77  (via drill 0.6)
  Sig1 0.406: R21.2 R23.2 72.07,87.31 71.75,87.63 U$13.1 71.75,91.44 71.12,92.08 v68.58,92.08
  Bottom 0.406: v68.58,92.08 C63.2
N$78  (via drill 0.6)
  Sig1 0.254: U$19.39 19.22,32.88 18.73,32.38 v18.73,31.43
  Bottom 0.254: R45.1 v18.73,31.43
N$79  (via drill 0.6)
  Sig1 0.406: v64.77,92.08 R24.1 R28.1
  Bottom 0.406: X23.1 63.5,93.66 63.82,93.34 64.45,93.34 64.77,93.03 v64.77,92.08
N$80  (via drill 0.6)
  Sig1 0.406: R24.2 R28.2 60.64,87.31 60.33,87.63 U$14.1 60.33,91.44 59.69,92.08 v57.15,92.08
  Bottom 0.406: v57.15,92.08 C58.2
N$81  (via drill 0.6)
  Sig1 0.254: U$19.40 19.99,32.38 19.68,32.07 19.68,30.16 v18.73,29.21
  Bottom 0.254: R46.1 v18.73,29.21
N$82  (via drill 0.6)
  Sig1 0.406: v53.34,92.08 R29.1 R31.1
  Bottom 0.406: X24.1 52.07,93.66 52.39,93.34 53.02,93.34 53.34,93.03 v53.34,92.08
N$83  (via drill 0.6)
  Sig1 0.406: R29.2 R31.2 49.21,87.31 48.9,87.63 U$15.1 48.9,91.44 48.26,92.08 v45.72,92.08
  Bottom 0.406: v45.72,92.08 C59.2 47.62,92.08
N$84
  Sig1 0.254: U$19.43 21.98,30.88 21.59,30.48 21.59,28.26 19.68,26.35 17.46,26.35 17.14,26.67 R40.1
  Sig1 0.406: R40.1
N$85  (via drill 0.6)
  Sig1 0.406: R34.1 R32.1 v41.91,92.08
  Bottom 0.406: X25.1 40.64,93.66 40.96,93.34 41.59,93.34 41.91,93.03 v41.91,92.08
N$86  (via drill 0.6)
  Sig1 0.406: R32.2 R34.2 37.78,87.31 37.47,87.63 U$16.1 37.47,91.44 36.83,92.08 v34.29,92.08
  Bottom 0.406: v34.29,92.08 C64.2
N$87
  Sig1 0.254: R41.1 14.92,26.35 15.56,25.72 20,25.72 22.23,27.94 22.23,29.84 22.75,30.38 U$19.44
N$88  (via drill 0.6)
  Sig1 0.406: R37.1 R35.1 v30.48,92.08
  Bottom 0.406: v30.48,92.08 30.48,93.03 30.16,93.34 29.53,93.34 29.21,93.66 X26.1
N$89  (via drill 0.6)
  Sig1 0.406: R35.2 R37.2 26.35,87.31 26.04,87.63 U$17.1 26.04,91.44 25.4,92.08 v22.86,92.08
  Bottom 0.406: v22.86,92.08 C65.2
N$90
  Sig1 0.254: U$19.45 23.21,29.88 22.86,29.53 22.86,27.62 20.32,25.08 R42.1
  Sig1 0.406: R42.1
N$91  (via drill 0.6)
  Sig1 0.254: U$19.41 20.45,31.88 20.32,31.75 20.32,29.53 18.73,27.94 v18.73,27.3
  Bottom 0.254: R47.1 18.41,26.99 v18.73,27.3
N$92  (via drill 0.6)
  Sig1 0.254: U$19.42 21.21,31.38 20.95,31.11 20.95,28.89 v20,27.94
  Bottom 0.254: R48.1 19.37,24.77 20,25.4 v20,27.94
N$93  (via drill 0.6)
  Sig1 0.254: U$19.37 19.78,33.88 18.73,34.92 v18.73,35.88
  Bottom 0.254: R52.2 v18.73,35.88
N$94
  Sig1 0.254: R49.2 SPDLED.C
N$95
  Sig1 0.254: R50.2 LINKLED.C
N$96
  Sig1 0.254: R51.2 ACTLED.C
N$97  (via drill 0.6)
  Sig1 0.254: U$19.10 30.86,25.79 v30.8,25.72
  Bottom 0.254: v30.8,25.72 31.11,25.4 R54.2
  Bottom 0.406: R54.2
N$98  (via drill 0.6)
  Sig1 0.254: U$19.20 34.8,31.88 v35.24,31.43
  Bottom 0.254: v35.24,31.43 C51.2
N$99  (via drill 0.6)
  Sig1 0.254: C53.1 v33.98,38.1 | Q2.2 33.34,42.16 33.34,38.73 v33.98,38.1 | U$19.30 29.36,36.98 30.48,38.1 v33.97,38.1 v33.98,38.1
  Bottom 0.305: v33.98,38.1 33.98,45.08 32.7,46.35 29.52,46.35 R55.2
N$100  (via drill 0.6)
  Sig1 0.254: C52.1 v23.18,38.41 23.81,39.05 23.81,42.23 Q2.1 | U$19.31 28.86,37.76 v29.53,38.42
  Bottom 0.254: v29.53,38.42 v23.18,38.42 v23.18,38.41
  Bottom 0.305: v23.18,38.41 23.18,44.77 24.77,46.35 27.31,46.35 R55.1
N$101
  Sig1 0.254: X27.6 20.32,16.83 22.54,19.05 29.53,19.05 30.16,19.68 R58.1 | R58.1 R59.2 | R58.1 31.11,20.95 31.43,21.27 31.43,21.59 31.75,21.91 C54.1
N$103
  Sig1 0.406: U$3.9 57.8,21.92 57.15,21.27 51.12,21.27 50.48,21.91 C66.2
N$104
  Sig1 0.254: X27.3 20.64,13.02 23.18,15.56 R60.1
N$105
  Sig1 0.406: U$4.9 83.52,21.92 82.87,21.27 81.92,21.27 81.28,20.64 81.28,20 80.96,19.68 79.06,19.68 C67.2
N$106
  Sig1 0.406: C68.2 106.23,19.55 108.6,21.92 U$5.9
N$107
  Sig1 0.406: U$8.9 94.94,49.86 94.3,49.21 89.53,49.21 C69.2
N$108
  Sig1 0.305: 115.57,49.05 C70.2
  Sig1 0.406: U$7.9 117.49,49.86 116.68,49.05 115.57,49.05
N$109
  Sig1 0.406: U$6.9 133.04,21.92 131.44,20.32 129.54,20.32 129.22,20 C71.2
N$110  (via drill 0.6)
  Sig1 0.406: U$24.1 46.67,10.79 46.35,10.48 46.04,10.48 45.72,10.79 v45.72,12.06
  Bottom 0.254: 45.4,9.84
  Bottom 0.406: 45.4,9.84 R4.2 45.72,10.47 v45.72,12.06 | C72.2 49.53,8.26 48.9,8.89 48.9,9.84 48.26,10.16 46.99,10.16 R7.2 45.41,9.84 45.4,9.84
RXN
  Sig1 0.254: U$19.5 28.36,23.6 R59.1 | R59.1 17.46,23.5 16.51,22.54 X27.8
  Sig1 0.406: R59.1 28.36,23.6
RXP
  Sig1 0.254: U$19.6 28.86,25.43 29.21,25.08 29.21,22.54 28.89,22.23 28.57,22.23 28.26,21.91 R58.2 | R58.2 | R58.2 25.08,20.96 24.45,21.59 20,21.59 19.05,20.64 X27.7
SPDLED  (via drill 0.6)
  Sig1 0.254: R49.1 17.14,35.24 17.78,35.88 17.78,36.2 18.41,36.83 19.37,36.83 19.68,36.51 19.68,34.61 20,34.29 23.18,34.29 v23.81,34.92 | v29.21,33.97 31.75,33.97 31.85,33.88 U$19.24
  Bottom_GND 0.254: v23.81,34.92 26.35,34.92 27.62,33.66 28.89,33.66 v29.21,33.97
SPI_CHAIN  (via drill 0.6)
  Sig1 0.406: U$5.25 124.97,19.96 125.57,19.37 127,19.37 127.16,19.53 127.16,21.11 v126.84,21.43 | U$6.27 149.53,21.26 v149.86,21.59
  Bottom_GND 0.254: 149.54,21.27 149.56,21.26
  Bottom_GND 0.406: v149.86,21.59 149.54,21.27 | v126.84,21.43 127.48,21.43 128.27,20.64 133.03,20.64 133.99,19.68 136.21,19.68 137.78,21.26 149.56,21.26
SPI_CLOCK  (via drill 0.6)
  Sig1 0.406: U$6.26 150.16,20.62 v151.13,21.59 153.99,24.45 153.99,27.3 151.76,29.53 151.76,36.51 151.13,37.15 146.05,37.15 144.15,39.05 144.15,47.94 141.92,50.16 139.7,50.16 139.06,49.53 137.79,49.53 137.48,49.21 v137.16,49.21 136.51,48.56 U$7.26 | U$3.26 75.23,20.62 v75.56,20.32 | U$8.26 112.54,48.56 113.35,49.37 v113.35,50.01 | U$4.26 98.48,20.64 99.85,20.64 100.17,20.32 v101.28,20.32 | U$5.26 123.88,20.64 125.09,20.64 125.25,20.48 125.41,20.48 125.57,20.32 v126.21,20.32
  Bottom_GND 0.406: v75.56,20.32 81.6,20.32 82.55,19.37 95.89,19.37 96.52,20 100.97,20 v101.28,20.32 104.78,20.32 105.09,20 108.27,20 108.58,19.68 125.41,19.68 v126.21,20.32 127.64,20.32 127.95,20 132.72,20 133.67,19.05 136.53,19.05 138.11,20.64 150.18,20.64 v151.13,21.59 | v137.16,49.21 123.83,49.21 120.65,52.39 117.47,52.39 115.09,50.01 v113.35,50.01
SPI_SDI  (via drill 0.6)
  Sig1 0.254: U$2.22 40.3,57.77 v40.96,58.42
  Sig1 0.406: U$3.27 75.23,21.26 v75.56,21.59 | v65.72,43.81 65.72,41.91 68.9,38.73 72.71,38.73 76.83,34.61 v76.83,31.11
  Sig2 0.406: v76.83,31.11 76.83,22.86 v75.56,21.59
  Bottom_GND 0.406: v40.96,58.42 40.96,49.21 42.55,47.62 59.37,47.62 62.23,44.77 63.18,44.77 63.82,44.13 65.41,44.13 v65.72,43.81
SPI_SDO  (via drill 0.6)
  Sig1 0.254: U$2.21 39.22,58.27 v40.01,59.05
  Sig1 0.406: U$8.25 113.31,47.9 v113.51,48.1
  Sig2 0.406: v113.51,48.1 113.35,47.94 98.74,47.94 94.3,43.5 v94.3,42.86
  Bottom_GND 0.406: v40.01,59.05 40.01,49.21 42.23,46.99 59.05,46.99 61.91,44.13 62.87,44.13 64.14,42.86 v94.3,42.86
TXN  (via drill 0.6)
  Sig1 0.254: U$19.1 26.36,26.36 v25.4,25.72 | X27.2 21.91,11.75 23.5,13.34 26.35,13.34 26.67,13.02 v27.94,13.02 R57.1
  Bottom_GND 0.254: v25.4,25.72 27.3,25.72 27.62,25.4 27.62,13.34 v27.94,13.02
TXP  (via drill 0.6)
  Sig1 0.254: R56.1 v26.67,10.48 25.4,10.48 25.08,10.79 22.86,10.79 22.54,10.48 X27.1 | U$19.2 26.86,24.96 v26.67,24.77
  Sig1 0.406: R56.1
  Bottom_GND 0.254: v26.67,10.48 v26.67,24.77
UART_ARM_RX
  Sig1 0.305: IC2.12 23.81,75.88 24.45,76.52 27.62,76.52 28.57,75.56 28.57,71.44 29.53,70.48 32.07,70.48 33.34,69.22 33.34,60.64 33.72,60.27 U$2.17
UART_ARM_TX
  Sig1 0.305: IC2.11 25.08,70.48 25.72,69.85 31.75,69.85 32.38,69.22 32.7,68.9 32.7,60.33 33.26,59.77 U$2.18
UART_PC_RX
  Sig1 0.61: X16.2 20.84,76 21.27,75.56 IC2.14
UART_PC_TX
  Sig1 0.61: IC2.13 22.54,75.56 21.27,76.83 17.78,76.83 16.83,77.79 16.83,78.42 16.51,78.74 X16.3
V+  (via drill 0.6)
  Sig1 0.406: U$3.16 54.7,17.37 v54.61,17.46 | U$3.15 55.33,18.01 v54.61,18.73 | U$3.4 55.02,25.17 v54.61,24.77 | U$3.5 55.63,24.51 v54.61,23.5 | U$6.4 130.26,25.17 v129.86,24.77 | U$6.5 130.87,24.51 v129.86,23.5 | U$8.4 92.8,53.11 v92.39,52.7 | U$8.5 93.41,52.45 v92.39,51.44 | U$7.16 117.39,45.31 v116.68,44.61 113.67,44.61 112.33,45.95 U$8.22 | U$7.15 116.77,45.95 v116.68,45.88 113.35,45.88 112.62,46.61 U$8.23 | U$8.16 92.64,45.31 v92.39,45.56 | U$8.15 93.28,45.95 v92.39,46.83 | U$3.34 75.97,25.81 76.52,26.35 76.52,27.62 77.47,28.57 79.06,28.57 v79.69,29.21 | U$3.33 76.29,25.17 77.15,26.04 77.15,27.3 77.79,27.94 v79.69,27.94 | U$4.34 101.05,25.81 101.6,26.35 101.6,27.94 102.71,29.05 104.3,29.05 v105.09,29.84 | U$4.33 101.37,25.17 102.23,26.04 102.23,27.62 103.03,28.42 v105.09,28.42 | U$3.22 76.29,18.01 78.42,15.88 v79.69,15.88 81.19,17.37 U$4.16 | 74.55,18.67 U$3.23 76.58,18.67 78.11,17.14 v79.69,17.14 80.56,18.01 U$4.15 | U$7.23 138.68,46.61 v139.7,47.62 | U$7.34 139.29,53.75 v139.7,53.34 | U$7.33 138.66,53.11 v139.7,52.07 | U$6.34 151.85,25.81 v152.72,26.67 | D3.1 C27.1 | C27.1 | C31.1 D5.1 C31.1 113.35,36.51 112.71,37.15 111.44,37.15 110.81,36.51 v110.81,35.88 | D6.1 C33.1 137.79,36.2 137.16,36.83 135.89,36.83 135.25,36.2 v135.25,35.88 | D8.1 C37.1 v97.47,62.87 | D7.1 C35.1 122.87,62.86 122.56,62.55 122.56,60.64 122.24,60.33 v121.28,60.33 | C29.1 D4.1 C29.1 87.95,36.2 87.31,36.83 86.04,36.83 85.41,36.2 v85.41,35.88 | v60.33,35.88 60.33,36.2 60.96,36.83 62.55,36.83 63.18,36.2 C27.1 | U$5.34 126.14,25.81 126.68,26.35 126.68,26.99 128.27,28.57 129.22,28.57 v129.86,29.21 | U$5.33 126.45,25.17 127.32,26.04 127.32,26.67 128.59,27.94 v129.86,27.94
  Sig1 0.406: U$7.22 139.29,45.95 v139.7,46.35 | U$7.4 118.18,53.11 v116.68,54.61 115.89,55.4 113.67,55.4 112.01,53.75 U$8.34 | U$7.5 117.73,52.45 v116.68,53.5 115.57,54.45 113.51,54.45 112.17,53.11 U$8.33 | U$4.4 82.46,25.17 82.23,25.4 v79.69,25.4 | U$4.5 80.07,24.51 v79.69,24.13 | U$6.33 152.49,25.17 v152.72,25.4 | U$6.22 152.49,18.01 v152.72,17.78 | U$6.23 152.34,18.67 v152.72,19.05 | U$5.4 108.18,25.17 107.95,25.4 v105.09,25.4 | U$5.5 105.47,24.51 v105.09,24.13 | U$4.22 102.01,18.01 103.5,16.51 v105.09,16.51 105.96,17.37 U$5.16 | U$4.23 102.3,18.67 103.19,17.78 v105.09,17.78 105.32,18.01 U$5.15 | U$5.22 126.77,18.01 128.91,15.88 v129.86,15.88 131.36,17.37 U$6.16 | U$6.15 130.72,18.01 v129.86,17.14 128.59,17.14 127.06,18.67 U$5.23
  Sig1 1.27: v139.7,47.62 141.6,47.62 142.88,46.35 v142.88,35.88
  Sig2 0.406: v92.39,52.7 93.66,53.66 95.25,53.66 95.89,54.29 95.89,58.1 97.47,59.69 v97.47,62.87 | v121.28,60.33 117.79,60.33 115.57,58.1 115.57,55.72 v116.68,54.61
  Sig2 1.27: v54.61,17.46 v54.61,18.73 v54.61,23.5 v54.61,24.77 54.61,31.11 56.83,33.34 56.83,35.88 | v79.69,15.88 v79.69,17.14 v79.69,24.13 v79.69,25.4 v79.69,27.94 v79.69,29.21 79.69,35.88 | v105.09,16.51 v105.09,17.78 v105.09,24.13 v105.09,25.4 v105.09,28.42 v105.09,29.84 105.09,35.88 | v129.86,15.88 v129.86,17.14 v129.86,23.5 v129.86,24.77 v129.86,27.94 v129.86,29.21 129.86,35.88 | v92.39,52.7 v92.39,51.44 v92.39,46.83 v92.39,45.56 92.39,35.88 | v116.68,54.61 v116.68,53.5 v116.68,45.88 v116.68,44.61 116.68,35.88 | v152.72,17.78 v152.72,19.05 v152.72,25.4 v152.72,26.67 152.72,35.88 | v139.7,53.34 v139.7,52.07 v139.7,47.62 v139.7,46.35
  Sig2 2.54: 154.62,35.88 X28.2
  Sig2 6.452: 154.62,35.88 152.72,35.88 v142.88,35.88 v135.25,35.88 129.86,35.88 116.68,35.88 v110.81,35.88 105.09,35.88 92.39,35.88 v85.41,35.88 79.69,35.88 v60.33,35.88 56.83,35.88
VCC  (via drill 0.6)
  Sig1 0.254: U$2.56 U$2.25 33.91,56.26 32.7,57.47 v31.11,57.47
  Bottom 0.254: v31.11,57.47 31.11,52.7 30.48,52.07 C8.1 29.21,52.07 | C16.1 30.32,54.45 30.48,54.61 30.48,56.83 | C15.1 30.48,56.83 | 30.48,56.83 v31.11,57.47 | C14.1 30.64,59.21 31.11,58.74 v31.11,57.47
